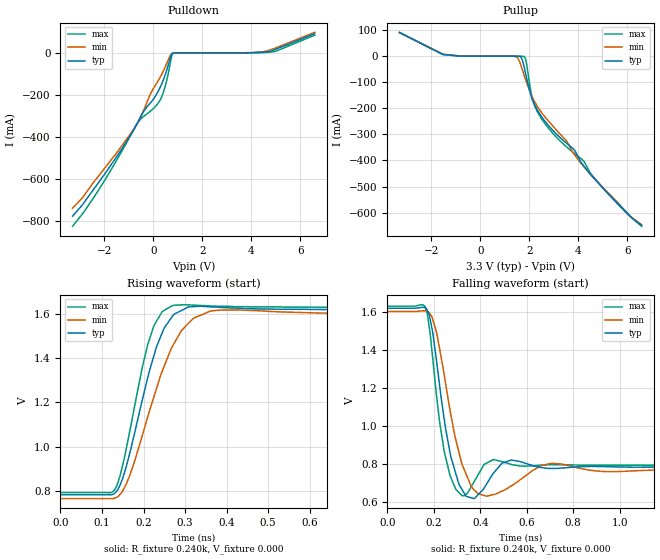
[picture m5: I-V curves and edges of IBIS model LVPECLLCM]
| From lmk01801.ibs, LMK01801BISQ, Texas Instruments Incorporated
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|   Model LVPECLLCM
[Model]   LVPECLLCM
Model_type   Output
Polarity   Non-Inverting
Vmeas = 1.15
Vref = 0
Cref = .3pF
Rref = 240
|   typ   min   max
|   (nom PVT)   (fast PVT)   (slow PVT)
C_comp   0.2109p   0.1807p   0.2310p
|C_comp (Low state)   0.2109p   0.1807p   0.2310p
|C_comp (High state)   0.9933p   0.9197p   1.0724p
[Voltage Range]   3.3   3.135   3.465
[Temperature Range]   45   125   -40
[Pullup Reference]   3.3   3.135   3.465
[Pulldown Reference]   0   0   0
[Power Clamp Reference]   3.3   3.135   3.465
[GND Clamp Reference]   0   0   0
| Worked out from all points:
|   slope of the pulldown table from 0 to 0.495 V, typ, clamps not added: 4.12 ohm
|   falling waveform, R_fixture 0.240k, V_fixture 0.000: 20-80 % time 56.4ps typ, 72.7ps min, 46.4ps max; typ from 1.62 V to 0.782 V
|   rising waveform, R_fixture 0.240k, V_fixture 0.000: 20-80 % time 67.2ps typ, 86.5ps min, 55.1ps max; typ from 0.782 V to 1.62 V
[Pulldown]
|   Voltage   I(typ)   I(min)   I(max)
-3.3V     -777.5mA   -739.6mA   -825.6mA
-2.062V   -589.1mA   -560.4mA   -621.1mA
-686.4mV  -341.5mA   -344.3mA   -340.1mA
-409.2mV  -281.7mA   -277.3mA   -303.2mA
-87.45mV  -234mA     -189.1mA   -274.4mA
283.8mV   -163.2mA   -115.6mA   -224.2mA
496.6mV   -100.5mA   -64.24mA   -154.1mA
749.1mV   -8.139mA   -4.51mA    -16.18mA
808.5mV   -1.36mA    -1.063mA   -1.493mA
4.516V    3.273mA    5.472mA    1.302mA
4.991V    16.56mA    23.05mA    6.859mA
6.595V    91.54mA    97.73mA    84.24mA
[Pullup]
|   Voltage   I(typ)   I(min)   I(max)
-3.3V     90.83mA    89.82mA    91.78mA
-1.503V   6.622mA    7.623mA    5.798mA
1.393V    -432.7nA   -252uA     -20.98nA
1.67V     -4.47mA    -36.71mA   -3.155uA
1.808V    -47.31mA   -76.94mA   -1.933mA
1.883V    -78.66mA   -97.55mA   -22.72mA
2.125V    -164.7mA   -155.9mA   -163.5mA
2.501V    -231.1mA   -215.8mA   -239.3mA
3.526V    -333.8mA   -325.1mA   -347.7mA
3.887V    -364.8mA   -382.5mA   -375.9mA
4.471V    -449.1mA   -449.8mA   -444.4mA
6.595V    -649.1mA   -646.1mA   -652.4mA
[Ramp]
R_load = 240
|   typ   min   max
dV/dt_r   0.487852/6.71966e-11   0.484778/8.64351e-11   0.491273/5.51589e-11
dV/dt_f   0.496836/5.63308e-11   0.496427/9.47887e-11   0.4979/4.64128e-11
[Falling Waveform]
R_fixture = 0.240k
V_fixture = 0.000
V_fixture_min = 0.000
V_fixture_max = 0.000
C_fixture = 0.000
|  time   V(typ)   V(min)   V(max)
0s        1.618V     1.601V     1.629V
162.1ps   1.621V     1.605V     1.628V
195.1ps   1.494V     1.56V      1.359V
244.7ps   1.035V     1.269V     865.2mV
321.5ps   663.9mV    796mV      631.2mV
374.6ps   615.1mV    660.2mV    706.4mV
456.4ps   748.8mV    636.5mV    821.4mV
533.5ps   818.9mV    682.1mV    795.4mV
707.4ps   774.4mV    801.4mV    794.1mV
1.999ns   781.6mV    764.3mV    791.6mV
[Rising Waveform]
R_fixture = 0.240k
V_fixture = 0.000
V_fixture_min = 0.000
V_fixture_max = 0.000
C_fixture = 0.000
|  time   V(typ)   V(min)   V(max)
0s        781.6mV    764.3mV    791.6mV
130.6ps   788.6mV    766.6mV    805mV
144ps     828.5mV    784.6mV    870.5mV
166.4ps   966.9mV    866.8mV    1.065V
209.9ps   1.309V     1.133V     1.46V
244.7ps   1.513V     1.339V     1.61V
269.9ps   1.59V      1.454V     1.638V
321.5ps   1.633V     1.582V     1.64V
390.8ps   1.629V     1.618V     1.635V
1.999ns   1.618V     1.601V     1.629V
